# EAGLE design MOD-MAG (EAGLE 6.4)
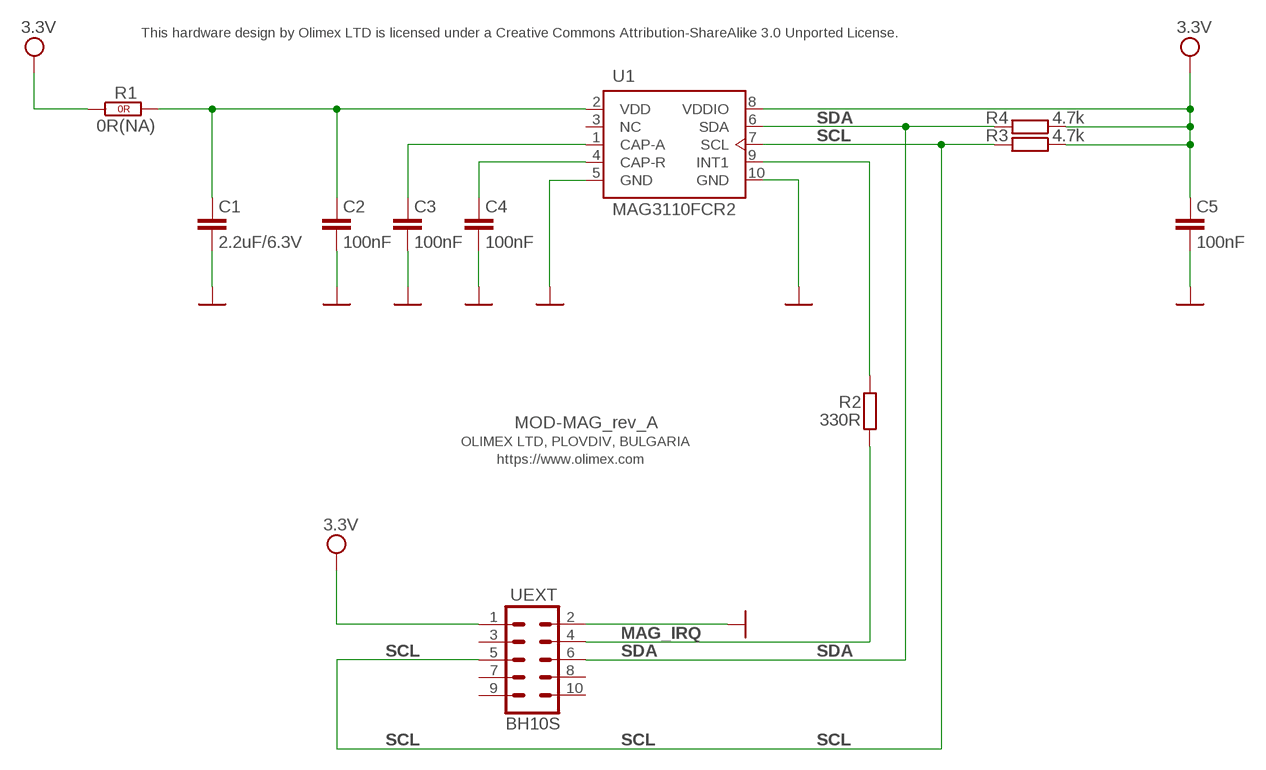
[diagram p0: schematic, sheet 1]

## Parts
C1  2.2uF/6.3V  C-EUC0603_DWS  [C0603_DWS]
C2  100nF  C-EUC0603_DWS  [C0603_DWS]
C3  100nF  C-EUC0603_DWS  [C0603_DWS]
C4  100nF  C-EUC0603_DWS  [C0603_DWS]
C5  100nF  C-EUC0603_DWS  [C0603_DWS]
R1  0R(NA)  R_0R0R(NA)  [0603_0R]
R2  330R  R-EU_R0603_5MIL_DWS  [R0603_5MIL_DWS]
R3  4.7k  R-EU_R0603_5MIL_DWS  [R0603_5MIL_DWS]
R4  4.7k  R-EU_R0603_5MIL_DWS  [R0603_5MIL_DWS]
U1  MAG3110FCR2  [DQFN10]
UEXT  BH10S  ML10SMD  [ML10_PADS]

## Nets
GND [PWR]: C1.2 C2.2 C3.2 C4.2 C5.2 U1.5(GND) U1.10(GND) UEXT.2
MAG_IRQ: R2.2 UEXT.4
MAG_VDD: C1.1 C2.1 R1.2(1.2) U1.2(VDD)
N$1: C3.1 U1.1(CAP-A)
N$2: C4.1 U1.4(CAP-R)
N$3: R2.1 U1.9(INT1)
SCL: R3.2 U1.7(SCL) UEXT.5
SDA: R4.2 U1.6(SDA) UEXT.6
VCC: C5.1 R1.1(1.1) R3.1 R4.1 U1.8(VDDIO) UEXT.1 ; supply symbol labelled 3.3V
Unconnected: U1.3(NC) UEXT.3 UEXT.7 UEXT.8 UEXT.9 UEXT.10

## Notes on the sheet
- This hardware design by Olimex LTD is licensed under a Creative Commons Attribution-ShareAlike 3.0 Unported License.
- MOD-MAG_rev_A
- OLIMEX LTD, PLOVDIV, BULGARIA
- https://www.olimex.com

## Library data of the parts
C1-C5 = rcl:C-EU: CAPACITOR, European symbol
R1 = OLIMEX_DISCRET:R_0R
R2-R4 = rcl:R-EU_: RESISTOR, European symbol
U1 = OLIMEX_IC:MAG3110
UEXT = con-harting-ml:ML10: HARTING

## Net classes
0 default: width 0.203 mm, drill 0.584 mm, clearance 0.178 mm
1 PWR: width 0.203 mm, drill 0.584 mm, clearance 0.178 mm

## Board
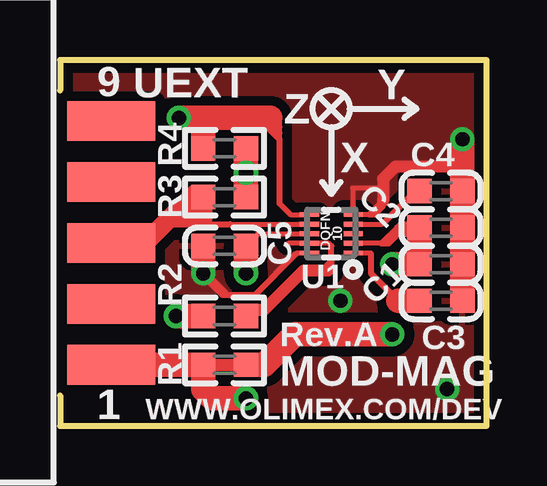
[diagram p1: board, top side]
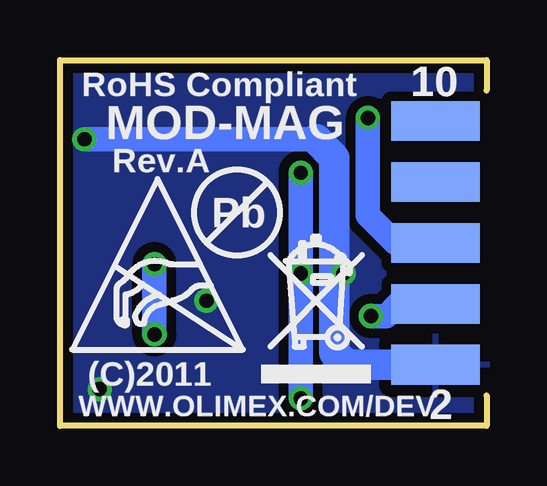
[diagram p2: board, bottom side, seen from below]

Size 17.78 x 15.24 mm. Coordinates in mm from the lower left corner, seen from the top.
Outline: 0,13.97 0,15.24 17.78,15.24 17.78,0 0,0 0,1.27
Copper layers (1+16): Top 0.035mm / dielectric 1.5mm / Bottom 0.035mm
Design rules "default": minimum track width 8mil, minimum drill 23mil, track to track 8mil, track to pad 8mil, pad to pad 8mil, via to via 10mil, smd to smd 1mil, copper to edge 10mil, drill to drill 8mil, minimum pad ring 10mil, minimum via ring 8mil, stop-mask expansion 4mil, vias tented up to drill 25mil, thermal gap 20mil

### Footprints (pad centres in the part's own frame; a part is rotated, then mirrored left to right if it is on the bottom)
C0603_DWS = smd 1.016 x 1.016: 1 -0.889,0; 2 0.889,0
0603_0R = smd 1.016 x 1.016: 1 -0.889,0; 2 0.889,0
R0603_5MIL_DWS = smd 1.016 x 1.016: 1 -0.889,0; 2 0.889,0
DQFN10 = smd 0.2 x 0.8: 1 -0.8,-0.91; 2 -0.4,-0.91; 3 0,-0.91; 4 0.4,-0.91; 5 0.8,-0.91; 6 0.8,0.91; 7 0.4,0.91; 8 0,0.91; 9 -0.4,0.91; 10 -0.8,0.91
ML10_PADS = smd 1.651 x 3.683: 1 -5.08,-0.229; 3 -2.54,-0.229; 5 0,-0.229; 7 2.54,-0.229; 9 5.08,-0.229 | smd 1.651 x 3.683 bottom: 2 -5.08,-0.229; 4 -2.54,-0.229; 6 0,-0.229; 8 2.54,-0.229; 10 5.08,-0.229

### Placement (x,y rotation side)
C1  15.88,6.73 0 top
C2  15.88,8.26 0 top
C3  15.88,5.21 0 top
C4  15.88,9.78 0 top
C5  6.86,7.49 180 top
R1  6.86,2.54 0 top
R2  6.86,4.57 180 top
R3  6.86,9.53 180 top
R4  6.86,11.56 180 top
U1  11.3,8 90 top
U$1  [ESD_SYMBOL]  17.27,3.17 0 bottom
U$3  [PB_SMALL]  10.41,8.89 0 bottom
U$4  [RECYCLE_BIN1/8]  9.4,1.78 0 bottom
UEXT  1.91,7.62 90 top

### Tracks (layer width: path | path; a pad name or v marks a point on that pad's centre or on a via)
GND  (via drill 0.6)
  Top 0.203: U1.10 9.87,7.2 9.83,7.16 | 12.99,8.8 13.12,8.8 13.46,9.14 13.46,9.27 | 12.87,8.8 12.99,8.8 | 12.87,8.8 U1.5 12.19,8.8 12.19,9.91 13.46,9.91 | 13.46,9.37 13.46,9.27 | 12.99,8.8 13.46,9.27 | 13.46,9.4 12.87,8.8
  Top 0.254: 9.83,7.16 8.13,5.46 6.86,5.46 6.78,5.54
  Top 0.406: v5.97,6.35 6.78,5.54
  Top 0.508: 13.46,9.37 13.46,9.4 13.46,9.91 13.46,10.29 13.97,10.79 16.76,10.79
  Top 1.016: v5.97,6.35 C5.2 | v16.76,11.94 16.76,10.79 C4.2 C2.2 C1.2 C3.2
  Bottom 1.016: 6.35,6.35 v5.97,6.35 | 7.11,11.94 v16.76,11.94
  Bottom 1.27: UEXT.2 5.84,2.54 6.35,3.05 6.35,6.35 6.35,11.18 7.11,11.94
  other vias: 11.68,5.21 16.13,1.52
  pour Bottom (isolate 0.406): 0,15.88 0,-0.64 18.41,-0.64 18.41,15.88
  pour Top (isolate 0.406): -0.64,16.51 -0.64,-1.27 19.05,-1.27 19.05,16.51
MAG_IRQ  (via drill 0.6)
  Top 1.016: v4.83,4.57 R2.2
  Bottom 1.016: v4.83,4.57 4.19,4.57 3.68,5.08 UEXT.4
MAG_VDD  (via drill 0.6)
  Top 0.203: 13.39,7.6 U1.2
  Top 0.254: 14.22,8.26 14.05,8.26 13.39,7.6 13.7,7.6 14.1,8 14.94,8
  Top 0.508: C2.1 14.22,8.26
  Top 1.016: C2.1 C1.1 v13.84,6.73 | R1.2 8.51,2.54 9.78,3.81 v13.84,3.81
  Bottom 1.016: v13.84,3.81 v13.84,6.73
N$1
  Top 0.203: U1.1 12.95,7.2 12.95,7.16
  Top 0.254: 12.95,7.16 12.95,6.35 14.1,5.21
  Top 1.016: 14.1,5.21 C3.1
N$2
  Top 0.203: U1.4 13.43,8.4 13.46,8.43
  Top 0.254: 13.46,8.43 14.81,9.78 C4.1
N$3
  Top 0.203: 10.43,7.6 11.2,7.6 11.3,7.49 | 10.43,7.6 U1.9 | 10.43,7.6 9.5,7.6
  Top 0.254: 11.3,6.86 11.3,6.6 11.18,6.48 | 11.3,6.86 11.3,7.49 | 10.92,6.48 11.3,6.86
  Top 0.508: 11.18,6.48 10.92,6.48 10.16,6.48 8.51,4.83 8,4.83 R2.1
SCL
  Top 0.203: 7.09,8.4 U1.7
  Top 0.254: 5.97,8.64 6.2,8.4 7.09,8.4
  Top 0.762: UEXT.5 3.56,7.62 4.57,8.64 | 4.57,8.64 5.97,8.64 R3.2 | 4.57,8.64 5.59,9.65 5.84,9.65
SDA  (via drill 0.6)
  Top 0.203: U1.6 9.61,8.8 9.14,9.27
  Top 0.254: 9.14,12.19 9.14,12.45 | 9.14,11.94 9.14,12.19 | 9.14,11.94 9.14,9.27 | 9.14,12.45 8.76,12.83 9.14,12.83 9.14,12.45 | 8.51,12.83 9.14,12.19 | 8.26,12.83 9.14,11.94
  Top 1.016: 5.97,12.83 8.26,12.83 8.51,12.83 8.76,12.83 | v4.95,12.83 5.97,12.83 | 5.97,12.83 R4.2
  Bottom 1.016: UEXT.6 3.81,7.62 4.95,8.76 v4.95,12.83
VCC  (via drill 0.6)
  Top 0.203: U1.8 8.26,8 C5.1
  Top 1.016: R4.1 v7.75,10.54 R3.1 | v7.75,6.35 C5.1 | v7.75,1.14 6.35,1.14 5.97,1.52 R1.1 UEXT.1
  Bottom 1.016: v7.75,10.54 v7.75,6.35 v7.75,1.14

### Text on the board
tNames: Z | Y | X | Rev.A | MOD-MAG | WWW.OLIMEX.COM/DEV
bNames: RoHS Compliant | MOD-MAG | Rev.A | (C)2011 | WWW.OLIMEX.COM/DEV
